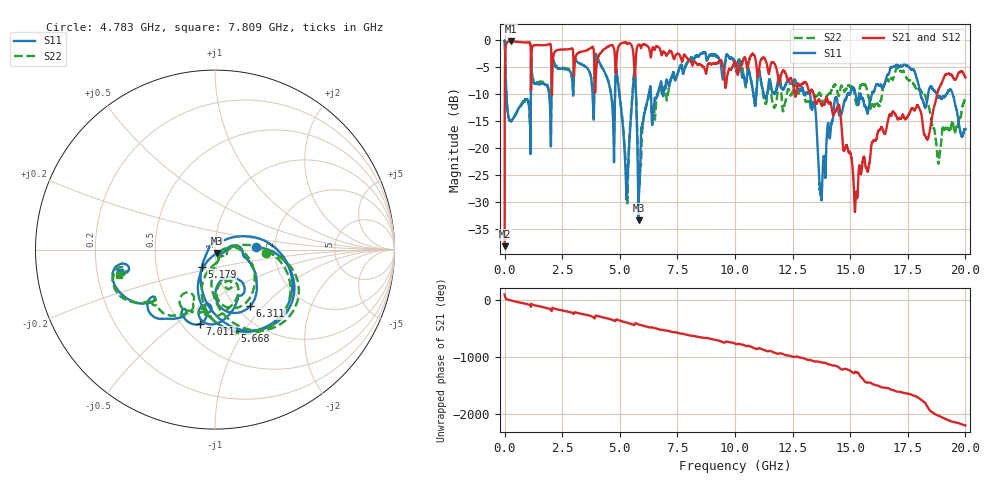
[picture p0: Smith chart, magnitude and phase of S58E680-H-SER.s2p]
!{S58E680}
!Johanson Technology Inc.
!www.johansontechnology.com
!Test Board Conditions:
!Substrate Type  RO4350B
!Substrate Thickness  60 mil
!Substrate Dk  3.66
!TL Type: GCPW
!TL Trace Width  115 mil
!TL Gap  52 mil
!Electrode orientation  Horizontal
!DUT TOPOLOGY	SERIES
!Mounting Pad LxW  55x428 mil
! Created Wed Apr 14 11:59:57 2021
# mhz S ma R 50
! 2 Port Network Data from SP1.SP block
! freq  magS11  angS11  magS21  angS21  magS12  angS12  magS22  angS22
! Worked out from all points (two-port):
!   20001 points, 300 kHz to 20 GHz, reference 50 ohm
!   highest |S21| = -0.20 dB at 287.3 MHz (marker M1); lowest = -38.1 dB at 300 kHz (marker M2)
!   |S21| within 3 dB of the highest: 23.47 MHz to 1.139 GHz (1.115 GHz wide, 192 % of centre); 5.698 GHz to 7.321 GHz (1.622 GHz wide, 24.9 % of centre)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
!   lowest |S11| = -33.3 dB at 5.817 GHz (marker M3), VSWR 1.04, Z = 51.1 - j1.89 ohm
!   |S11| at or under -10 dB: 78.09 MHz to 1.137 GHz (1.059 GHz wide, 174 % of centre); 4.985 GHz to 5.552 GHz (567.6 MHz wide, 10.8 % of centre); 13.26 GHz to 14.88 GHz (1.615 GHz wide, 11.5 % of centre)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
!   |S22| runs from -30.2 to 0.0 dB; largest |S21 - S12| = 0.0067
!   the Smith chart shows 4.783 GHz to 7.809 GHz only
!   S11 on the Smith chart (normalised r, x): 4.783 GHz: 1.59, +0.05; 5.179 GHz: 0.85, -0.16; 5.668 GHz: 0.79, -0.91; 6.311 GHz: 1.16, -0.84; 7.011 GHz: 0.61, -0.61; 7.809 GHz: 0.30, -0.11
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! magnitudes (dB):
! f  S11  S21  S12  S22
! 300 kHz  0.0  -38.1  -38.0  0.0
! 105.3 MHz  -11.9  -0.4  -0.4  -11.9
! 287.3 MHz  -14.9  -0.2  -0.2  -15.0
! 3.334 GHz  -4.4  -2.1  -2.1  -4.4
! 4.783 GHz  -12.8  -2.8  -2.8  -10.9
! 5.179 GHz  -18.4  -0.4  -0.4  -17.9
! 5.326 GHz  -26.7  -0.7  -0.7  -30.1
! 5.668 GHz  -6.6  -5.8  -5.8  -6.4
! 5.817 GHz  -33.3  -0.8  -0.8  -23.2
! 6.311 GHz  -8.6  -2.2  -2.2  -9.2
! 6.667 GHz  -9.5  -1.2  -1.2  -9.7
! 7.011 GHz  -7.5  -2.8  -2.8  -9.6
! 7.809 GHz  -5.3  -2.6  -2.6  -5.2
! 10 GHz  -4.4  -3.9  -3.9  -4.7
! 13.33 GHz  -12.7  -9.2  -9.1  -12.6
! 13.72 GHz  -28.5  -11.7  -11.7  -10.2
! 14.36 GHz  -10.6  -13.2  -13.2  -8.3
! 15.25 GHz  -10.3  -28.5  -28.7  -11.5
! 16.67 GHz  -6.2  -14.3  -14.6  -7.5
! 18.34 GHz  -11.2  -18.3  -18.4  -11.5
! 18.84 GHz  -10.6  -9.0  -9.1  -22.5
! 20 GHz  -16.4  -6.9  -6.8  -11.2
